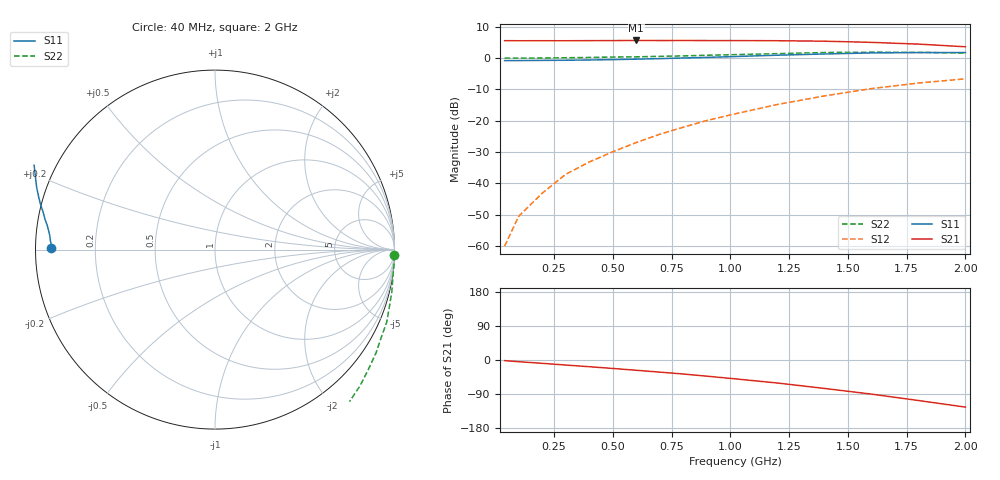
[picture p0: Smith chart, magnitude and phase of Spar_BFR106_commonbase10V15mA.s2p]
! Filename:  BFR106CE.S2P  Version:  2.0
! NXP part #: BFR106  Date: Jul 1990
! Bias condition: Vce=10V, Ic=15mA
! COMMON BASE
#  MHz  S  MA  R  50
! Freq  S11  S21  S12  S22
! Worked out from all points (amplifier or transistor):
!   16 points, 40 MHz to 2 GHz, reference 50 ohm
!   highest |S21| = 5.6 dB at 600 MHz (marker M1)
!   |S21| within 3 dB of that: start of sweep to end of sweep
!   unconditionally stable (mu >= 1): nowhere
!   at 200 MHz: K = -0.55, MSG = 24.3 dB, |S12| = -43.1 dB
!   at 800 MHz: K = -0.90, MSG = 13.8 dB, |S12| = -22.0 dB
!   at 2 GHz: K = -0.69, MSG = 5.1 dB, |S12| = -6.6 dB
40  0.911 179.4  1.895 -1.7  0.001 77.4  0.999 -1.8
100  0.913 178.1  1.891 -4.5  0.003 100.5  1.001 -4.5
200  0.919 176.8  1.892 -8.8  0.007 121.0  1.003 -9.0
300  0.924 175.1  1.891 -13.3  0.014 129.7  1.013 -13.5
400  0.933 173.5  1.896 -17.7  0.022 134.1  1.023 -18.3
500  0.945 171.7  1.901 -22.3  0.032 136.7  1.039 -23.0
600  0.962 169.9  1.911 -27.1  0.045 137.7  1.047 -27.7
700  0.98 167.7  1.904 -32.0  0.061 138.7  1.066 -32.7
800  1.004 165.5  1.907 -37.0  0.079 139.1  1.084 -37.9
900  1.026 163.3  1.903 -42.7  0.101 137.6  1.109 -43.3
1000  1.053 160.7  1.902 -48.5  0.124 135.4  1.131 -48.5
1200  1.112 155.0  1.892 -60.7  0.182 130.3  1.178 -60.5
1400  1.163 148.0  1.86 -75.0  0.249 123.1  1.227 -73.1
1600  1.209 140.1  1.782 -90.0  0.326 115.3  1.241 -86.7
1800  1.224 131.3  1.671 -106.9  0.4 105.7  1.236 -101.2
2000  1.226 123.2  1.516 -124.3  0.467 96.7  1.199 -115.7
